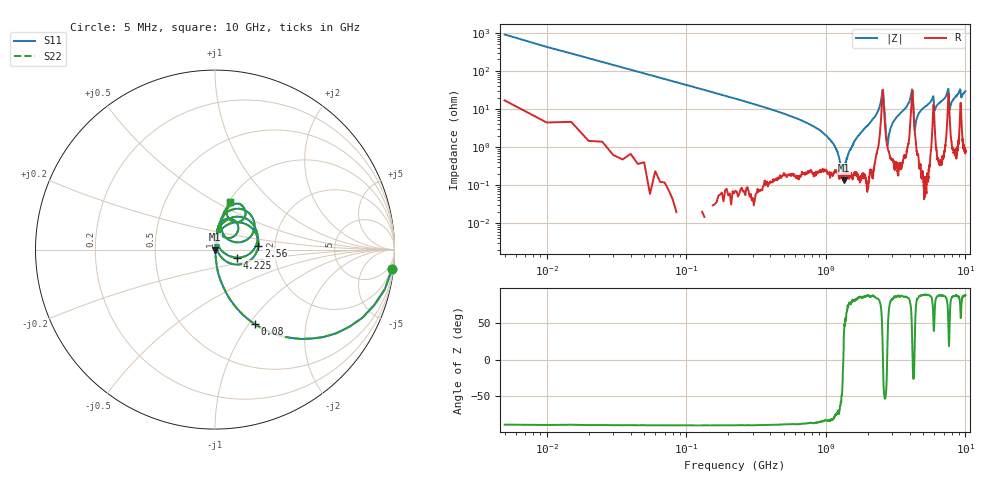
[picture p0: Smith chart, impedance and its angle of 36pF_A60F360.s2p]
! Amotech Co.,Ltd.
! http://www.amotech.co.kr/
! Part Number: A60F360
! These Parameters are Measured in Series Mode Connection
! Operation Temp=25[degC], DC Bias Voltage=0[V]
! Freq. Start=5[MHz] Stop=10[GHz], 2000[Steps]
! Date: Monday, July 20, 2020, 04:19:15
# GHZ S RI R 50.000000
!Freq.(Hz) S11(Real) S11(Imag) S21(Real) S21(Imag) S12(Real) S12(Imag) S22(Real) S22(Imag)
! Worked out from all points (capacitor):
!   2000 points, 5 MHz to 10 GHz, reference 50 ohm
!   read as one part in series: C = 36.9 pF near 55 MHz
!   lowest |Z| = 135 mohm at 1.34 GHz (marker M1)
!   series resonance near 1.336 GHz, so ESL is about 380 pH
!   S11 on the Smith chart (normalised r, x): 5 MHz: 1, -18; 80 MHz: 1.00, -1.07; 2.56 GHz: 1.64, +0.07; 4.225 GHz: 1.27, -0.12; 10 GHz: 1.02, +0.59
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0.005  0.986 -0.1088  0.014 0.1088  0.014 0.1088  0.986 -0.1088
0.08  0.2236 -0.4162  0.7764 0.4162  0.7764 0.4162  0.2236 -0.4162
0.315  0.0172 -0.1277  0.9828 0.1277  0.9828 0.1277  0.0172 -0.1277
1.1  0.00223 -0.0139  0.9978 0.0139  0.9978 0.0139  0.00223 -0.0139
1.34  0.00134 0.000199  0.9987 -0.000199  0.9987 -0.000199  0.00134 0.000199
1.675  0.00226 0.0179  0.9977 -0.0179  0.9977 -0.0179  0.00226 0.0179
2.56  0.242 0.0215  0.758 -0.0215  0.758 -0.0215  0.242 0.0215
2.765  0.01 0.00396  0.99 -0.00396  0.99 -0.00396  0.01 0.00396
3  0.00625 0.0404  0.9938 -0.0404  0.9938 -0.0404  0.00625 0.0404
3.34  0.00834 0.0692  0.9917 -0.0692  0.9917 -0.0692  0.00834 0.0692
4.125  0.1893 0.162  0.8107 -0.162  0.8107 -0.162  0.1893 0.162
4.225  0.1212 -0.045  0.8788 0.045  0.8788 0.045  0.1212 -0.045
4.35  0.0221 0.0161  0.9779 -0.0161  0.9779 -0.0161  0.0221 0.0161
4.595  0.0113 0.0708  0.9887 -0.0708  0.9887 -0.0708  0.0113 0.0708
5.005  0.0126 0.1053  0.9874 -0.1053  0.9874 -0.1053  0.0126 0.1053
5.845  0.0905 0.1705  0.9095 -0.1705  0.9095 -0.1705  0.0905 0.1705
6.02  0.0425 0.0752  0.9575 -0.0752  0.9575 -0.0752  0.0425 0.0752
6.67  0.0276 0.15  0.9724 -0.15  0.9724 -0.15  0.0276 0.15
7.515  0.1895 0.2034  0.8105 -0.2034  0.8105 -0.2034  0.1895 0.2034
7.725  0.0568 0.0708  0.9432 -0.0708  0.9432 -0.0708  0.0568 0.0708
8.335  0.0432 0.1838  0.9568 -0.1838  0.9568 -0.1838  0.0432 0.1838
10  0.085 0.2657  0.915 -0.2657  0.915 -0.2657  0.085 0.2657
